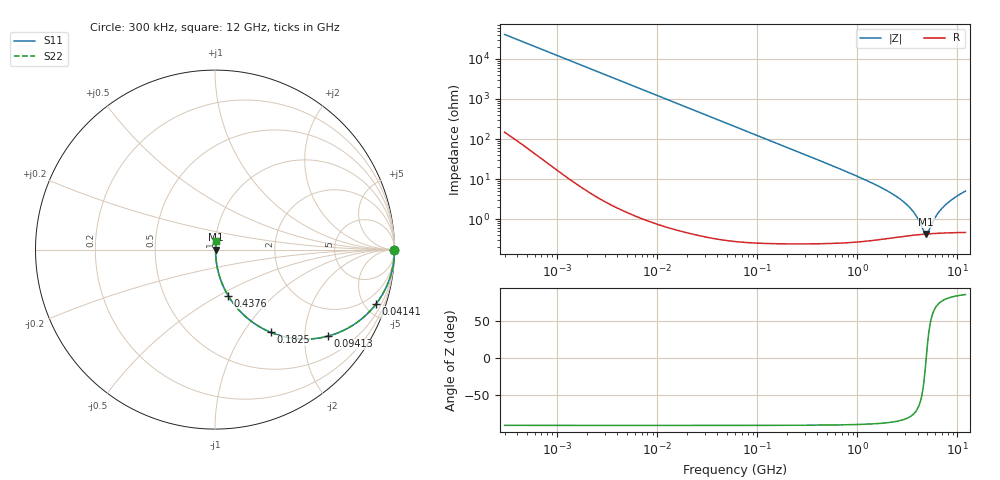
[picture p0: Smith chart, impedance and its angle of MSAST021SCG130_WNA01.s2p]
! MSAST021SCG130_WNA01  S-PARAMETER MODEL  ( Standard Model )
! Model Generated by TAIYO YUDEN Corporation (http://www.ty-top.com)
! Version 1.0
! TAIYO YUDEN Control No. 241126
! Copyright(c) 2024 TAIYO YUDEN CO.,LTD. All Rights Reserved.
! Product Description (link to TY-COMPAS)
! https://ds.yuden.co.jp/TYCOMPAS/or/detail?pn=MSAST021SCG130JWNA01&u=M
! Products Name : Multilayer Ceramic Capacitors
! Characteristics :
!  Capacitance : 13 [pF] , Rated Voltage : 25 [V] , TCC : CG / C0G
!  Case Size : 0.25 x 0.125 / 0.0098 x 0.0049 [mm/inch] , Thickness : 0.125 / 0.0049 [mm/inch]
!  (Conditions: Temperature = 25 [degC] , DC Bias Voltage = 0 [V])
! External Node Assignments :
!  1  o---| |---o  2
! GND o---------o GND
! Frequency Range : 0.3MHz  -  12000MHz  [ 401 STEP ]
# MHZ S RI R 50
! Freq[MHz].  S11 Real  S11 Imag  S21 Real  S21 Imag  S12 Real  S12 Imag  S22 Real  S22 Imag
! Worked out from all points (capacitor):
!   401 points, 300 kHz to 12 GHz, reference 50 ohm
!   read as one part in series: C = 13 pF near 316.3 kHz
!   lowest |Z| = 423 mohm at 4.875 GHz (marker M1)
!   series resonance near 4.875 GHz, so ESL is about 82 pH
!   S11 on the Smith chart (normalised r, x): 300 kHz: open; 41.41 MHz: 1.01, -5.93; 94.13 MHz: 1.01, -2.61; 182.5 MHz: 1.00, -1.34; 437.6 MHz: 1.00, -0.56; 12 GHz: 1.01, +0.10
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0.3  1 -0.00245  1.49e-05 0.00245  1.49e-05 0.00245  1 -0.00245
1.769972  0.9998 -0.0144  0.000221 0.0144  0.000221 0.0144  0.9998 -0.0144
10.44266  0.9928 -0.0845  0.00725 0.0845  0.00725 0.0845  0.9928 -0.0845
21.35258  0.9705 -0.1689  0.0295 0.1689  0.0295 0.1689  0.9705 -0.1689
41.40751  0.8975 -0.3028  0.1025 0.3028  0.1025 0.3028  0.8975 -0.3028
60  0.8067 -0.3943  0.1933 0.3943  0.1933 0.3943  0.8067 -0.3943
94.13233  0.6291 -0.4821  0.3709 0.4821  0.3709 0.4821  0.6291 -0.4821
182.544  0.3112 -0.4612  0.6888 0.4612  0.6888 0.4612  0.3112 -0.4612
353.9943  0.1078 -0.3067  0.8922 0.3067  0.8922 0.3067  0.1078 -0.3067
437.5599  0.0736 -0.2568  0.9264 0.2568  0.9264 0.2568  0.0736 -0.2568
1105.905  0.0135 -0.1029  0.9865 0.1029  0.9865 0.1029  0.0135 -0.1029
2088.533  0.00551 -0.0468  0.9945 0.0468  0.9945 0.0468  0.00551 -0.0468
2722.03  0.00453 -0.0301  0.9955 0.0301  0.9955 0.0301  0.00453 -0.0301
3364.605  0.0042 -0.0185  0.9958 0.0185  0.9958 0.0185  0.0042 -0.0185
3944.255  0.00414 -0.0104  0.9959 0.0104  0.9959 0.0104  0.00414 -0.0104
4623.766  0.00418 -0.00257  0.9958 0.00257  0.9958 0.00257  0.00418 -0.00257
4875.354  0.00422 1.81e-06  0.9958 -1.81e-06  0.9958 -1.81e-06  0.00422 1.81e-06
5140.631  0.00426 0.00256  0.9957 -0.00256  0.9957 -0.00256  0.00426 0.00256
6026.253  0.00447 0.0103  0.9955 -0.0103  0.9955 -0.0103  0.00447 0.0103
7064.448  0.00479 0.0183  0.9952 -0.0183  0.9952 -0.0183  0.00479 0.0183
8966.534  0.00552 0.0311  0.9945 -0.0311  0.9945 -0.0311  0.00552 0.0311
12000  0.00706 0.0492  0.9929 -0.0492  0.9929 -0.0492  0.00706 0.0492
